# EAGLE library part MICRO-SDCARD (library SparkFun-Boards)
microSD Card Footprint This is the mechnical footprint with connections for soldering a microSD card - NOT for a socket for the card. SparkFun Products: MicroSD Card with Adapter - 8 GB
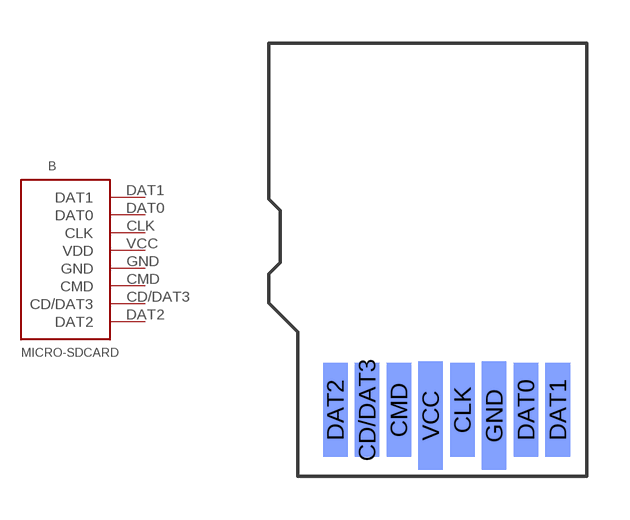
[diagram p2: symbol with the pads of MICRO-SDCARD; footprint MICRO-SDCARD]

Designator prefix B

## MICRO-SDCARD  [MICRO-SDCARD]
CD/DAT3  CD/DAT3
CLK  CLK
CMD  CMD
DAT0  DAT0
DAT1  DAT1
DAT2  DAT2
GND  GND
VCC  VDD

## Footprint MICRO-SDCARD (pad centres in mm)
smd 0.85 x 3.25 bottom: CD/DAT3 2.56,2.3; CLK 5.86,2.3; CMD 3.66,2.3; DAT0 8.06,2.3; DAT1 9.16,2.3; DAT2 1.46,2.3
smd 0.85 x 3.75 bottom: GND 6.96,2.1; VCC 4.76,2.1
